[IBIS ver]   4.2
[File name]   tm4c129cncpdt_128qfp_v0p0.ibs
[File Rev]   v0p0
[Date]   Sep 17, 2013
[Source]   simulation
[Notes]   IBIS models for 128qfp package with updated GPIO models
[Disclaimer] Please be aware that in the absence of a written agreement,
   Texas Instruments (TI) assumes no liability for: 1) the
   accuracy of the IBIS models provided to your company, 2) the
   proper functioning of these IBIS models in your design or for
   any resulting applications, or; 3) infringement of patents,
   copyrights, or intellectual property rights resulting from
   your use of these IBIS models. TI provides IBIS models as a
   service to our customers and therefore reserves the right to
   limit distribution of the IBIS models.
   This preliminary model does not contain all of the possible pad
   models for each of the pad types.  The most commonly used modes
   have been provided and the next update will include all of the
   pad model combinations.
   The only missing model that needs to be highlighted is the
   model for the USB D+ and D- GPIOs.  Currently only the USB
   functionality is provided on the D+ and D- pins.  Customers
   needing to model the PGIOs associated with these pins should
   check for a newer model.
[Copyright]   Property of Texas Instruments Incorporated. Unauthorized
   reproduction and/or distribution is strictly prohibited. This
   product is protected under copyright law and trade secret law
   as an unpublished work. Copyright (C) 2013, Texas Instruments
   Incorporated, all rights reserved. These commodities are under
   the U.S. Government distribution license control. As such,
   they are not to be re-exported without the prior approval of
   the U.S. Department of Commerce.
|   Component TM4C129CNCPDT
[Component]   TM4C129CNCPDT
[Manufacturer]   Texas Instruments Inc.
[Package]
| 128-pin QFP
| variable   typ   min   max
R_Pkg   2.49E-01   2.14E-01   2.82E-01
L_pkg   5.35E-09   4.77E-09   5.93E-09
C_pkg   1.18E-12   1.05E-13   1.46E-12
[Pin]   signal_name   model_name   R_pin   L_pin   C_pin
1   PD0   GPIO12P   2.74716E-01   5.67591E-09   1.25496E-12
2   PD1   GPIO12P   2.66097E-01   5.70179E-09   1.44936E-12
3   PD2   GPIO12P   2.58431E-01   5.64204E-09   1.40706E-12
4   PD3   GPIO12P   2.51716E-01   5.64216E-09   1.36344E-12
5   PQ0   GPIO12P   2.46023E-01   5.49459E-09   1.32209E-12
6   PQ1   GPIO12P   2.41580E-01   5.43987E-09   1.28280E-12
7   VDD   POWER
8   VDDA   POWER
9   VREFAP   NC
10   GNDA   GND
11   PQ2   GPIO12P   2.39002E-01   5.26478E-09   1.09382E-12
12   PE3   GPIO12P   2.38350E-01   5.20682E-09   1.05463E-12
13   PE2   GPIO12P   2.39188E-01   5.16972E-09   1.03340E-12
14   PE1   GPIO12P   2.40396E-01   5.12864E-09   1.01865E-12
15   PE0   GPIO12P   2.42832E-01   5.13151E-09   1.01581E-12
16   VDD   POWER
17   GND   GND
18   PK0   GPIO12P   2.47050E-01   5.21890E-09   9.99433E-13
19   PK1   GPIO12P   2.48989E-01   5.30666E-09   1.02924E-12
20   PK2   GPIO12P   2.52063E-01   5.39211E-09   1.05019E-12
21   PK3   GPIO12P   2.55225E-01   5.46691E-09   1.06544E-12
22   PC7   GPIO12P   2.57453E-01   5.49735E-09   1.11011E-12
23   PC6   GPIO12P   2.60269E-01   5.53816E-09   1.18111E-12
24   PC5   GPIO12P   2.64977E-01   5.67491E-09   1.20974E-12
25   PC4   GPIO12P   2.69639E-01   5.72206E-09   1.25424E-12
26   VDD   POWER
27   PQ3   GPIO12P   2.78218E-01   5.93356E-09   1.28923E-12
28   VDD   POWER
29   PH0   GPIO12P   2.57695E-01   5.55133E-09   1.35709E-12
30   PH1   GPIO12P   2.64238E-01   5.55399E-09   1.41108E-12
31   PH2   GPIO12P   2.72435E-01   5.61466E-09   1.45934E-12
32   PH3   GPIO12P   2.81711E-01   5.49509E-09   1.27221E-12
33   PA0   GPIO12P   2.65187E-01   5.47082E-09   1.24148E-12
34   PA1   GPIO12P   2.57430E-01   5.48532E-09   1.43612E-12
35   PA2   GPIO12P   2.51020E-01   5.50312E-09   1.39402E-12
36   PA3   GPIO12P   2.45630E-01   5.51865E-09   1.35166E-12
37   PA4   GPIO12P   2.41511E-01   5.42948E-09   1.31391E-12
38   PA5   GPIO12P   2.38415E-01   5.31620E-09   1.28219E-12
39   VDD   POWER
40   PA6   GPIO12P   2.37474E-01   5.24203E-09   1.20654E-12
41   PA7   GPIO12P   2.36922E-01   5.24384E-09   1.18332E-12
42   PF0   GPIO12P   2.37158E-01   5.23178E-09   1.15936E-12
43   PF1   GPIO12P   2.39776E-01   5.25060E-09   1.10213E-12
44   PF2   GPIO12P   2.41742E-01   5.23063E-09   1.05955E-12
45   PF3   GPIO12P   2.45278E-01   5.27513E-09   1.03954E-12
46   PF4   GPIO12P   2.49056E-01   5.26123E-09   1.00056E-12
47   VDD   POWER
48   GND   GND
49   PG0   GPIO12P   2.46871E-01   5.08761E-09   9.62364E-13
50   PG1   GPIO12P   2.45111E-01   5.16055E-09   9.85470E-13
51   PG2   GPIO12P   2.46139E-01   5.18339E-09   9.87716E-13
52   PG3   GPIO12P   2.47333E-01   5.22932E-09   9.88379E-13
53   PG4   GPIO12P   2.48661E-01   5.25640E-09   9.91314E-13
54   PG5   GPIO12P   2.51951E-01   5.26932E-09   9.98493E-13
55   PG6   GPIO12P   2.53181E-01   5.31052E-09   1.05320E-13
56   PG7   GPIO12P   2.65112E-01   5.40123E-09   1.15115E-12
57   PQ5   GPIO12P   2.72111E-01   5.46055E-09   1.25229E-12
58   PQ6   GPIO12P   2.81721E-01   5.59519E-09   1.27211E-12
59   PK7   GPIO12P   2.38090E-01   5.29631E-09   1.29871E-12
60   PK6   GPIO12P   2.41432E-01   5.33392E-09   1.34325E-12
61   PK5   GPIO12P   2.45792E-01   5.36801E-09   1.38217E-12
62   PK4   GPIO12P   2.51233E-01   5.32888E-09   1.41152E-12
63   VDD   POWER
64   WAKE_n   WAKE_INPUT   2.52532E-01   5.07323E-09   1.22600E-12
65   HIB_n   HIB_OUTPUT   2.47544E-01   5.17772E-09   1.22443E-12
66   XOSC0   NC
67   XOSC1   NC
68   VBAT   POWER
69   VDD   POWER
70   RST_n   RST_INPUT   2.26920E-01   5.16868E-09   1.26202E-12
71   PM7   GPIO8P   2.22111E-01   5.01857E-09   1.22832E-12
72   PM6   GPIO8P   2.18394E-01   4.96618E-09   1.19143E-12
73   PM5   GPIO8P   2.15736E-01   4.89541E-09   1.15798E-12
74   PM4   GPIO8P   2.14081E-01   4.86187E-09   1.12024E-12
75   PM3   GPIO12P   2.15869E-01   4.86688E-09   1.04909E-12
76   PM2   GPIO12P   2.16409E-01   4.84225E-09   1.01871E-12
77   PM1   GPIO12P   2.16856E-01   4.80246E-09   1.00901E-12
78   PM0   GPIO12P   2.17893E-01   4.77260E-09   9.97856E-13
79   VDD   POWER
80   GND   GND
81   PL0   GPIO12P   2.23883E-01   4.81866E-09   9.44742E-13
82   PL1   GPIO12P   2.24503E-01   4.84692E-09   9.92477E-13
83   PL2   GPIO12P   2.26379E-01   4.88866E-09   1.00681E-12
84   PL3   GPIO12P   2.29391E-01   4.96853E-09   1.03082E-12
85   PL4   GPIO12P   2.32776E-01   5.03314E-09   1.06029E-12
86   PL5   GPIO12P   2.37466E-01   5.17256E-09   1.11106E-12
87   VDDC   POWER
88   OSC0   NC
89   OSC1   NC
90   VDD   POWER
91   PB2   GPIO12P   2.26371E-01   5.21576E-09   1.27693E-12
92   PB3   GPIO12P   2.32562E-01   5.29789E-09   1.30856E-12
93   PL7   USB_PHY_DM   2.38750E-01   5.38023E-09   1.33664E-12
94   PL6   USB_PHY_DP   2.43025E-01   5.38516E-09   1.37862E-12
95   PB0   GPIO8P_5V   2.50881E-01   5.36978E-09   1.42580E-12
96   PB1   GPIO8P_5V   2.58293E-01   5.33272E-09   1.23967E-12
97   PC3_TDO_SWO   GPIO12P   2.65955E-01   5.42973E-09   1.23851E-12
98   PC2_TDI   GPIO12P   2.60202E-01   5.51450E-09   1.42464E-12
99   PC1_TMS_SWDIO  GPIO12P   2.56766E-01   5.54194E-09   1.37915E-12
100   PC0_TCK_SWCLK  GPIO12P   2.54027E-01   5.52541E-09   1.34750E-12
101   VDD   POWER
102   PQ4   GPIO12P   2.65991E-01   5.83612E-09   1.27549E-12
103   PP2   GPIO12P   2.62731E-01   5.75213E-09   1.25678E-12
104   PP3   GPIO12P   2.60049E-01   5.68619E-09   1.22349E-12
105   PP4   GPIO12P   2.58145E-01   5.54450E-09   1.19137E-12
106   PP5   GPIO12P   2.56647E-01   5.48205E-09   1.15554E-12
107   PN0   GPIO12P   2.59709E-01   5.50975E-09   1.10156E-12
108   PN1   GPIO12P   2.58653E-01   5.44794E-09   1.06224E-12
109   PN2   GPIO12P   2.58743E-01   5.45067E-09   1.03866E-12
110   PN3   GPIO12P   2.58872E-01   5.44676E-09   1.02224E-12
111   PN4   GPIO12P   2.59871E-01   5.47792E-09   1.02003E-12
112   PN5   GPIO12P   2.61739E-01   5.54958E-09   9.86818E-13
113   VDD   POWER
114   GND   GND
115   VDDC   POWER
116   PJ0   GPIO2   2.57312E-01   5.42569E-09   1.05816E-12
117   PJ1   GPIO2   2.55383E-01   5.43365E-09   1.07518E-12
118   PP0   GPIO12P   2.54943E-01   5.47506E-09   1.11858E-12
119   PP1   GPIO12P   2.53943E-01   5.49458E-09   1.15707E-12
120   PB5   GPIO12P   2.52020E-01   5.47232E-09   1.17643E-12
121   PB4   GPIO12P   2.52655E-01   5.43893E-09   1.23050E-12
122   VDD   POWER
123   PE4   GPIO12P   2.53224E-01   5.42249E-09   1.28669E-12
124   PE5   GPIO12P   2.56033E-01   5.54028E-09   1.32918E-12
125   PD4   GPIO12P   2.59874E-01   5.63949E-09   1.36608E-12
126   PD5   GPIO12P   2.64889E-01   5.62521E-09   1.40743E-12
127   PD6   GPIO12P   2.70702E-01   5.60843E-09   1.44943E-12
128   PD7   GPIO12P   2.77870E-01   5.40957E-09   1.28901E-12
[Model Selector] GPIO12P
GPIO12P_I/O_2   2mA Output Buffer
GPIO12P_I/O_4   4mA Output Buffer
GPIO12P_I/O_8S   8mA Output Buffer with Slew Rate Control
GPIO12P_I/O_8   8mA Output Buffer
GPIO12P_I/O_12S   12mA Output Buffer with Slew Rate Control
GPIO12P_I/O_12   12mA Output Buffer
GPIO12P_I_WPU_2   2ma Input with Pull-Up
GPIO12P_I_WPD_2   2mA Input with Pull-Down
GPIO12P_I/O_OD_2   2mA Output Buffer with Open Drain
GPIO12P_I/O_OD_4   4mA Output Buffer with Open Drain
GPIO12P_I/O_OD_8S   8mA Output Buffer with Open Drain and Slew Rate Control
GPIO12P_I/O_OD_8   8mA Output Buffer with Open Drain
GPIO12P_I/O_OD_12S   12mA Output Buffer with Open Drain and Slew Rate Control
GPIO12P_I/O_OD_12   12mA Output Buffer with Open Drain
[Model Selector] GPIO8P
GPIO8P_I/O_2   2mA Output Buffer
GPIO8P_I/O_4   4mA Output Buffer
GPIO8P_I/O_8S   8mA Output Buffer with Slew Rate Control
GPIO8P_I/O_8   8mA Output Buffer
GPIO8P_I_WPU_2   2mA Input with Pull-Up
GPIO8P_I_WPD_2   2mA Input with Pull-Down
GPIO8P_I/O_OD_2   2mA Output Buffer with Open Drain
GPIO8P_I/O_OD_4   4mA Output Buffer with Open Drain
GPIO8P_I/O_OD_8S   8mA Output Buffer with Open Drain and Slew Rate Control
GPIO8P_I/O_OD_8   8mA Output Buffer with Open Drain
GPIO8P_I_TAMPER   Tamper Input Model
GPIO8P_I_TAMPER_VWPU   Tamper Input Model with Very Weak Pull-Up
[Model Selector] GPIO8P_5V
GPIO8P_5V_I/O_2   2mA Output Buffer
GPIO8P_5V_I/O_4   4mA Output Buffer
GPIO8P_5V_I/O_8S   8mA Output Buffer with Slew Rate Control
GPIO8P_5V_I/O_8   8mA Output Buffer
GPIO8P_5V_I_WPU_2   2mA Input with Pull-Up
GPIO8P_5V_I_WPD_2   2mA Input with Pull-Down
GPIO8P_5V_I/O_OD_2   2mA Output Buffer with Open Drain
GPIO8P_5V_I/O_OD_4   4mA Output Buffer with Open Drain
GPIO8P_5V_I/O_OD_8S   8mA Output Buffer with Open Drain and Slew Rate Control
GPIO8P_5V_I/O_OD_8   8mA Output Buffer with Open Drain
[Model Selector] GPIO2
GPIO2_I/O_2   2mA Output Buffer
GPIO2_I_WPU_2   2mA Input with Pull-Up
GPIO2_I_WPD_2   2mA Input with Pull-Down
GPIO2_I/O_OD_2   GPIO2_I/O_OD_2
[Model Selector] RST_INPUT
RESET_INPUT   Reset Pad Input Model
[Model Selector] HIB_OUTPUT
HIBERNATE_OUTPUT   Output Buffer for the HIB_n Pin
[Model Selector] WAKE_INPUT
WAKE_IN   Input Model for the WAKE_n Pin
[Model Selector] USB_PHY_DP
fsdp_tx   Full Speed transmitter--12Mbps
lsdp_50pf_tx   Low speed transmitter--1.5Mbps driving 50pF cap load
lsdp_200pf_tx   Low speed transmitter--1.5Mbps driving 200pF cap load
lsdp_400pf_tx   Low speed transmitter--1.5Mbps driving 400pF cap load
lsdp_600pf_tx   Low speed transmitter--1.5Mbps driving 600pF cap load
fsdp_rx   Recieve mode--Open circuit during fs/ls recieve mode
[Model Selector] USB_PHY_DM
fsdm_tx   Full Speed transmitter--12Mbps
lsdm_50pf_tx   Low speed transmitter--1.5Mbps driving 50pF cap load
lsdm_200pf_tx   Low speed transmitter--1.5Mbps driving 200pF cap load
lsdm_400pf_tx   Low speed transmitter--1.5Mbps driving 400pF cap load
lsdm_600pf_tx 	 Low speed transmitter--1.5Mbps driving 600pF cap load
fsdm_rx   Recieve mode--Open circuit during fs/ls recieve mode
| Models and submodels in the file (55): GPIO12P_I/O_2 (I/O), GPIO12P_I/O_4 (I/O), GPIO12P_I/O_8S (I/O), GPIO12P_I/O_8 (I/O), GPIO12P_I/O_12S (I/O), GPIO12P_I/O_12 (I/O), GPIO12P_I_WPU_2 (Input), GPIO12P_I_WPD_2 (Input), GPIO12P_I/O_OD_2 (I/O_open_drain), GPIO12P_I/O_OD_4 (I/O_open_drain), GPIO12P_I/O_OD_8S (I/O_open_drain), GPIO12P_I/O_OD_8 (I/O_open_drain), GPIO12P_I/O_OD_12S (I/O_open_drain), GPIO12P_I/O_OD_12 (I/O_open_drain), GPIO8P_I/O_2 (I/O), GPIO8P_I/O_4 (I/O), GPIO8P_I/O_8S (I/O), GPIO8P_I/O_8 (I/O), GPIO8P_I_WPU_2 (Input), GPIO8P_I_WPD_2 (Input), GPIO8P_I/O_OD_2 (I/O_open_drain), GPIO8P_I/O_OD_4 (I/O_open_drain), GPIO8P_I/O_OD_8S (I/O_open_drain), GPIO8P_I/O_OD_8 (I/O_open_drain), GPIO8P_I_TAMPER (Input), GPIO8P_I_TAMPER_VWPU (Input), GPIO8P_5V_I/O_2 (I/O), GPIO8P_5V_I/O_4 (I/O), GPIO8P_5V_I/O_8S (I/O), GPIO8P_5V_I/O_8 (I/O), GPIO8P_5V_I_WPU_2 (Input), GPIO8P_5V_I_WPD_2 (Input), GPIO8P_5V_I/O_OD_2 (I/O_open_drain), GPIO8P_5V_I/O_OD_4 (I/O_open_drain), GPIO8P_5V_I/O_OD_8S (I/O_open_drain), GPIO8P_5V_I/O_OD_8 (I/O_open_drain), GPIO2_I/O_2 (I/O), GPIO2_I_WPU_2 (Input), GPIO2_I_WPD_2 (Input), GPIO2_I/O_OD_2 (I/O_open_drain), RESET_INPUT (Input), HIBERNATE_OUTPUT (Output), WAKE_IN (Input), fsdp_tx (3-state), lsdp_50pf_tx (3-state), lsdp_200pf_tx (3-state), lsdp_400pf_tx (3-state), lsdp_600pf_tx (3-state), fsdp_rx (Input), fsdm_tx (3-state), lsdm_50pf_tx (3-state), lsdm_200pf_tx (3-state), lsdm_400pf_tx (3-state), lsdm_600pf_tx (3-state), fsdm_rx (Input)
